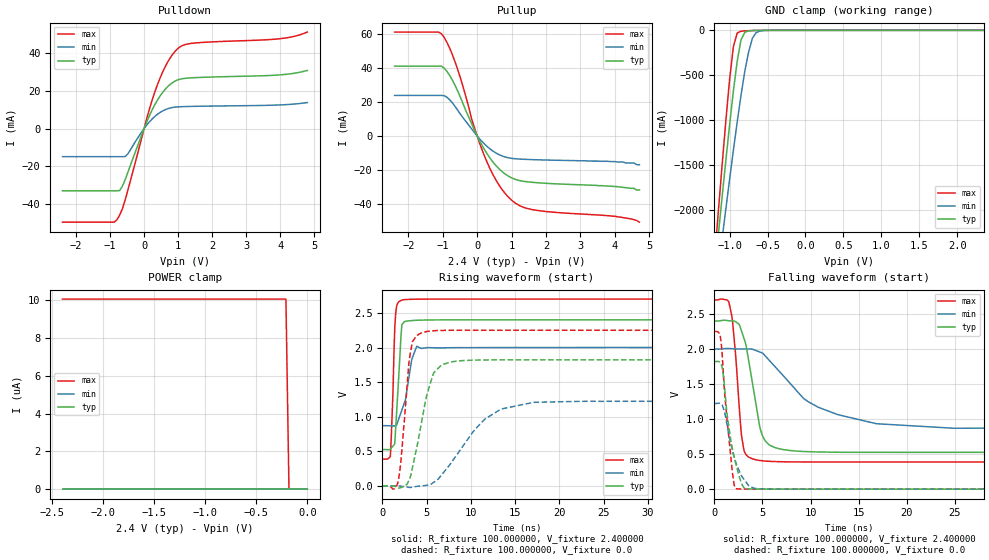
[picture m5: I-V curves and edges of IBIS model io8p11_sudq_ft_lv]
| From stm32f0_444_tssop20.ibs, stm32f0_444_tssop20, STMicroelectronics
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|   Model io8p11_sudq_ft_lv
[Model]  io8p11_sudq_ft_lv
Model_type I/O
Polarity   Non-Inverting
Enable   Active-Low
Vinl =   0.720000V
Vinh =   1.680000V
Vmeas =  1.200000V
Cref =   50.000000pF
Rref =   100.000000M
Vref =   0.0V
C_comp   1.970100pF   1.887900pF   2.069400pF
[Temperature Range]   25.000000   0.125000k   -40.000000
[Pullup Reference]   2.400000V   2.000000V   2.700000V
[Pulldown Reference]   0.0V   0.0V   0.0V
[POWER Clamp Reference]   2.400000V   2.000000V   2.700000V
[GND Clamp Reference]   0.0V   0.0V   0.0V
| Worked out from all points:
|   slope of the pulldown table from 0 to 0.36 V, typ, clamps not added: 25.5 ohm
|   slope of the pullup table from 0 to 0.36 V, typ, clamps not added: 28.4 ohm
|   GND clamp passes 1 mA (typ) near -0.64 V on its own axis
|   rising waveform, R_fixture 100.000000, V_fixture 2.400000: 20-80 % time 509ps typ, 1.05ns min, 338ps max; typ from 0.525 V to 2.4 V
|   rising waveform, R_fixture 100.000000, V_fixture 0.0: 20-80 % time 1.79ns typ, 4.5ns min, 865ps max; typ from 0 V to 1.82 V
|   falling waveform, R_fixture 100.000000, V_fixture 2.400000: 20-80 % time 1.38ns typ, 6.07ns min, 772ps max; typ from 2.4 V to 0.525 V
|   falling waveform, R_fixture 100.000000, V_fixture 0.0: 20-80 % time 1.17ns typ, 1.4ns min, 851ps max; typ from 1.82 V to 0 V
[Pulldown]
|Voltage   I(typ)   I(min)   I(max)
-2.4V     -33.16mA   -14.98mA   -49.86mA
-880mV    -33.16mA   -14.98mA   -49.86mA
-800mV    -33.16mA   -14.98mA   -48.55mA
-640mV    -30.75mA   -14.98mA   -42.76mA
-480mV    -23.43mA   -13.57mA   -32.92mA
80mV      3.651mA    1.905mA    5.506mA
400mV     15.37mA    7.665mA    23.73mA
720mV     22.75mA    10.69mA    36.23mA
1.04V     26.18mA    11.57mA    43.27mA
1.52V     27.09mA    11.81mA    45.55mA
4V        28.55mA    12.55mA    47.81mA
4.8V      30.9mA     13.81mA    51.31mA
[Pullup]
|Voltage   I(typ)   I(min)   I(max)
-2.4V     41.23mA    23.94mA    61.35mA
-1.12V    41.23mA    23.94mA    61.35mA
-960mV    40.07mA    23.8mA     58.26mA
-800mV    35.78mA    21.41mA    51.94mA
-560mV    26.31mA    15mA       38.91mA
-160mV    7.322mA    4.15mA     10.02mA
240mV     -8.977mA   -5.327mA   -13.21mA
640mV     -19.5mA    -11.09mA   -29.16mA
1.04V     -25.16mA   -13.38mA   -38.61mA
1.68V     -27.56mA   -14.07mA   -43.82mA
4V        -29.9mA    -15.2mA    -47.5mA
4.72V     -32mA      -17mA      -51mA
[GND_clamp]
|Voltage   I(typ)   I(min)   I(max)
-2.4V     -9.788A    -9.782A    -9.734A
-1.2V     -2.718A    -3.02A     -2.568A
-1.15V    -2.29A     -2.675A    -2.036A
-1.1V     -1.868A    -2.333A    -1.515A
-1.05V    -1.454A    -1.995A    -1.012A
-950mV    -674.5mA   -1.337A    -180.5mA
-900mV    -345.2mA   -1.023A    -29.72mA
-850mV    -106.4mA   -726mA     -10.13mA
-750mV    -6.396mA   -244mA     -4.026mA
-700mV    -2.558mA   -88.61mA   -2.329mA
-600mV    -416uA     -7.739mA   -368uA
2.35V     0A         0A         0A
[POWER_clamp]
|Voltage   I(typ)   I(min)   I(max)
-2.4V     0A         0A         10.06uA
-210mV    0A         0A         10.06uA
-180mV    0A         0A         0A
0V        0A         0A         0A
[Ramp]
| variable   typ   min   max
dV/dt_r  1.09302/1.79298n   0.73362/4.49721n   1.34964/0.86038n
dV/dt_f  1.12491/1.37677n   0.67799/6.06609n   1.38752/0.77139n
R_load = 100.000000
[Rising Waveform]
R_fixture= 100.000000
V_fixture= 2.400000
V_fixture_min= 2.000000
V_fixture_max= 2.700000
|time   V(typ)   V(min)   V(max)
0s        525.2mV    870.3mV    387.4mV
900.9ps   532.8mV    868.8mV    423.8mV
1.201ns   575.8mV    867.5mV    1.36V
1.401ns   611.9mV    867.1mV    2.288V
1.602ns   1.043V     877.1mV    2.592V
2.202ns   2.329V     1.096V     2.685V
2.603ns   2.378V     1.242V     2.693V
3.303ns   2.389V     1.815V     2.697V
3.904ns   2.394V     2.018V     2.698V
49.85ns   2.4V       2V         2.7V
[Rising Waveform]
R_fixture= 100.000000
V_fixture= 0.0
V_fixture_min= 0.0
V_fixture_max= 0.0
|time   V(typ)   V(min)   V(max)
0s        -34.42uV   -16.09uV   -30.78uV
1.802ns   -29.45mV   -740.6uV   67.32mV
3.103ns   111mV      -21.81mV   1.872V
3.403ns   265.9mV    -17.89mV   2.083V
4.505ns   973.7mV    1.595mV    2.215V
5.706ns   1.601V     43.39mV    2.241V
6.707ns   1.75V      161.3mV    2.247V
10.71ns   1.818V     849.4mV    2.249V
13.61ns   1.822V     1.116V     2.249V
49.85ns   1.822V     1.223V     2.249V
[Falling Waveform]
R_fixture= 100.000000
V_fixture= 2.400000
V_fixture_min= 2.000000
V_fixture_max= 2.700000
|time   V(typ)   V(min)   V(max)
0s        2.4V       2V         2.7V
1.502ns   2.403V     2.008V     2.671V
1.902ns   2.401V     2.004V     2.368V
2.903ns   2.223V     2.001V     690.6mV
4.004ns   1.477V     1.995V     431mV
5.205ns   706.9mV    1.914V     401.7mV
7.508ns   557.6mV    1.566V     389.5mV
10.81ns   530.8mV    1.169V     387.3mV
16.82ns   525.4mV    935mV      387.5mV
49.85ns   525.2mV    870.3mV    387.4mV
[Falling Waveform]
R_fixture= 100.000000
V_fixture= 0.0
V_fixture_min= 0.0
V_fixture_max= 0.0
|time   V(typ)   V(min)   V(max)
0s        1.822V     1.223V     2.249V
700.7ps   1.784V     1.214V     2.101V
1.101ns   1.383V     1.071V     1.306V
1.301ns   1.083V     925.1mV    1.011V
1.802ns   626.2mV    594.7mV    324.2mV
2.102ns   432.6mV    434mV      34.1mV
2.302ns   323.4mV    348.4mV    4.72mV
3.103ns   15.77mV    135.4mV    1.387mV
4.605ns   1.159mV    5.956mV    462.6uV
49.85ns   -34.42uV   -16.09uV   -30.78uV
